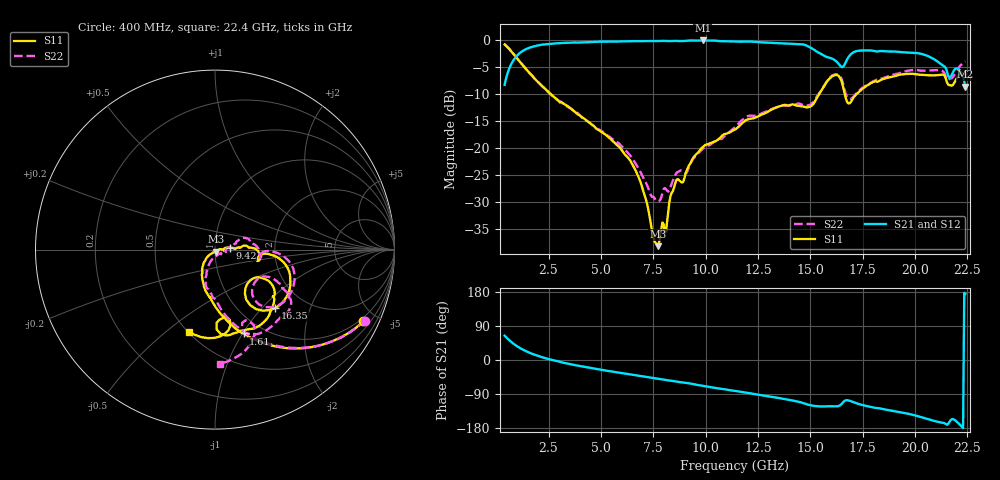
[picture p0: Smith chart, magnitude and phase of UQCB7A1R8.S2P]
!  Part Number  UQCB7A1R8	Mounting Orientation: Vertical
!  Description: RF capacitors
!  Application: Coupling, Bypass, Tuning, DC Block
!  Filters, Matching
# GHZ S DB R 50
! Freq  |S11|  S11 Ph  |S21|  S21 Ph  |S12|  S12 Ph  |S22|  S22 Ph
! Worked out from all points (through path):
!   401 points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, 400 MHz to 22.4 GHz, reference 50 ohm
!   highest |S21| = 0.00 dB at 9.86 GHz (marker M1); lowest = -8.6 dB at 22.4 GHz (marker M2)
!   group delay of S21, straight-line fit = 24.4 ps
!   lowest |S11| = -38.1 dB at 7.715 GHz (marker M3), VSWR 1.03, Z = 50.5 - j1.12 ohm
!   |S11| at or under -10 dB: 2.622 GHz to 15.41 GHz (12.79 GHz wide, 142 % of centre); 16.65 GHz to 17.19 GHz (542.7 MHz wide, 3.21 % of centre)
!   |S22| runs from -29.8 to -0.7 dB; largest |S21 - S12| = 0.0042
!   S11 on the Smith chart (normalised r, x): 400 MHz: 0.83, -4.21; 1.61 GHz: 0.82, -1.01; 9.42 GHz: 1.18, +0.03; 16.35 GHz: 1.43, -1.19; 22.4 GHz: 0.50, -0.60
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0.4  -0.74 -25.8  -8.23 64.3  -8.21 64.3  -0.69 -25.4
0.895  -2.85 -49.9  -3.27 40.1  -3.26 40.1  -2.80 -49.2
1.61  -6.14 -71.2  -1.31 18.6  -1.30 18.6  -6.13 -70.1
4.085  -14.19 -109.8  -0.36 -16.7  -0.35 -16.7  -14.26 -105.6
6.45  -22.61 -134.2  -0.14 -38.5  -0.13 -38.6  -21.59 -112.0
7.715  -38.13 -63.3  -0.11 -49.4  -0.11 -49.5  -29.82 -58.7
7.77  -37.57 -49.5  -0.10 -49.9  -0.11 -50.0  -29.79 -52.2
8.54  -26.56 0.2  -0.07 -56.4  -0.08 -56.5  -25.04 -12.0
9.42  -21.68 8.1  -0.01 -64.0  -0.01 -64.1  -21.87 9.2
9.86  -19.78 4.8  0.00 -67.9  -0.01 -68.0  -20.08 12.2
11.4  -16.51 6.0  -0.19 -81.7  -0.19 -81.8  -16.10 22.9
14.04  -11.95 -10.3  -0.61 -105.7  -0.62 -105.7  -12.03 -6.0
15.085  -12.00 -7.9  -1.51 -120.3  -1.51 -120.2  -11.61 -3.7
15.91  -7.07 -19.2  -3.19 -121.7  -3.23 -121.5  -6.95 -13.8
16.35  -6.60 -44.1  -4.35 -121.3  -4.35 -121.4  -6.37 -37.8
16.845  -11.69 -42.0  -2.94 -107.0  -2.95 -106.9  -10.82 -40.2
18.77  -6.84 -45.8  -2.04 -132.4  -2.04 -132.4  -6.56 -30.8
20.585  -6.42 -70.8  -2.86 -155.7  -2.86 -155.6  -5.58 -47.9
21.465  -7.03 -88.8  -5.11 -169.1  -5.12 -169.0  -6.62 -71.2
21.74  -8.37 -81.6  -6.45 -156.7  -6.47 -156.4  -7.02 -64.5
22.07  -6.50 -83.6  -5.29 -167.1  -5.28 -167.0  -5.07 -68.7
22.4  -6.33 -107.7  -8.59 174.3  -8.60 174.4  -3.92 -87.3
